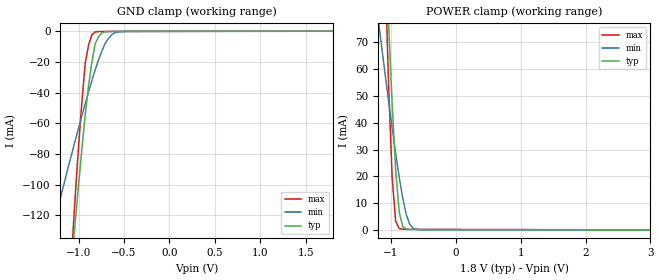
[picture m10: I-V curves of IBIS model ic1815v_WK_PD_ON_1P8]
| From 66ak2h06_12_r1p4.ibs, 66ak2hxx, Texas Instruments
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|   Model Cell ic1815v_WK_PD_ON_1P8
|WK_PD_ON_1P8
[Model]   ic1815v_WK_PD_ON_1P8
Model_type   Input
Polarity   Non-Inverting
Vinl =  0.63
Vinh =  1.17
C_comp   0.751145p   0.686962p   0.76914p
[Model Spec]
Vinl   0.63   0.567   0.693
Vinh   1.17   1.053   1.287
[Temperature Range]   25   125   -40
[Voltage Range]   1.8   1.62   1.98
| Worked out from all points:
|   GND clamp passes 1 mA (typ) near -0.74 V on its own axis
|   POWER clamp passes 1 mA (typ) near -0.80 V on its own axis
[POWER_clamp]
|   voltage   I(typ)   I(min)   I(max)
-1.8V     581.9mA    200.6mA    781mA
-1.182V   165.9mA    75.75mA    178.4mA
-1.073V   98.3mA     54.85mA    83.2mA
-1.055V   87.54mA    51.44mA    68.69mA
-1.036V   76.79mA    48.03mA    54.19mA
-981.8mV  47.16mA    38.12mA    19.77mA
-927.3mV  22.36mA    28.6mA     3.28mA
-872.7mV  6.638mA    19.73mA    499.3uA
-818.2mV  1.245mA    11.87mA    265.7uA
-763.6mV  295.4uA    5.734mA    246.9uA
-600mV    142.3uA    188.9uA    236.9uA
3.6V      0A         0A         0A
[GND_clamp]
|   voltage   I(typ)   I(min)   I(max)
-1.8V     -691.6mA   -252.4mA   -924.6mA
-1.291V   -306.2mA   -129.9mA   -367.2mA
-1.073V   -148.8mA   -79.28mA   -141.6mA
-1.036V   -123.7mA   -71.05mA   -106.5mA
-1V       -99.72mA   -62.98mA   -74.48mA
-927.3mV  -54.5mA    -47.17mA   -20.82mA
-890.9mV  -35.8mA    -39.62mA   -9.127mA
-854.5mV  -20.35mA   -32.3mA    -2.306mA
-818.2mV  -8.134mA   -25.22mA   -358.6uA
-709.1mV  -251.2uA   -7.977mA   -76.47uA
-563.6mV  -38.82uA   -434.4uA   -59.94uA
1.8V      111.5uA    64.31uA    177.9uA
